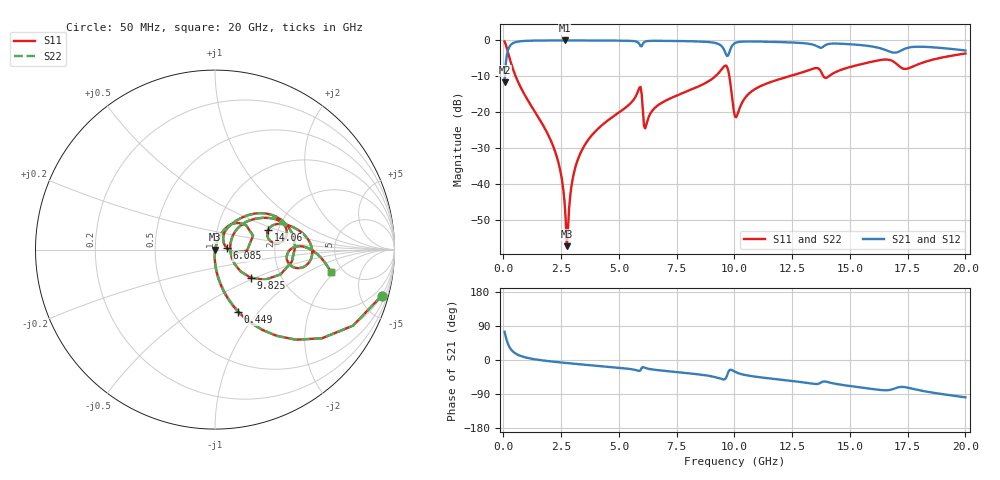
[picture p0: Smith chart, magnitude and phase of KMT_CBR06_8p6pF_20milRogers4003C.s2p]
! Data measured by Modelithics Inc. support@modelithics.com 813-866-6335
! KEMET CBR0603 8.6pF, Pad Width= 0.851mm, Pad Length= 0.64mm, Pad Gap= 0.62mm, 20mil Rogers 4003C substrate Data, January 2022
# hz S ma R 50
! 2 Port Network Data from SP1.SP block
! freq  magS11  angS11  magS21  angS21  magS12  angS12  magS22  angS22
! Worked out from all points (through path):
!   401 points, 50 MHz to 20 GHz, reference 50 ohm
!   highest |S21| = -0.01 dB at 2.643 GHz (marker M1); lowest = -11.6 dB at 50 MHz (marker M2)
!   group delay of S21, straight-line fit = 14.5 ps
!   lowest |S11| = -57.2 dB at 2.743 GHz (marker M3), VSWR 1.00, Z = 50.1 - j0.0686 ohm
!   |S11| at or under -10 dB: 530.9 MHz to 9.169 GHz (8.638 GHz wide, 178 % of centre); 9.781 GHz to 12.35 GHz (2.574 GHz wide, 23.3 % of centre); 13.86 GHz to 14.08 GHz (223.3 MHz wide, 1.6 % of centre)
!   |S22| runs from -57.2 to -0.3 dB; largest |S21 - S12| = 0
!   S11 on the Smith chart (normalised r, x): 50 MHz: 0.98, -7.27; 449 MHz: 0.98, -0.79; 6.085 GHz: 1.14, +0.02; 9.825 GHz: 1.40, -0.47; 14.06 GHz: 1.77, +0.42; 20 GHz: 4.01, -1.79
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5e7  0.9647 -15.4  0.2628 74.6  0.2628 74.6  0.9647 -15.4
2.495e8  0.5893 -54.5  0.8071 35.4  0.8071 35.4  0.5893 -54.5
4.49e8  0.3698 -69.5  0.9282 20.4  0.9282 20.4  0.3698 -69.5
2.194625e9  0.03114 -92.6  0.9983 -4.7  0.9983 -4.7  0.03114 -92.6
2.493875e9  0.01364 -91.4  0.9986 -6.6  0.9986 -6.6  0.01364 -91.4
2.6435e9  0.005742 -84.8  0.9986 -7.5  0.9986 -7.5  0.005742 -84.8
2.74325e9  0.001379 -29.8  0.9986 -8.1  0.9986 -8.1  0.001379 -29.8
3.0425e9  0.01397 74.7  0.9984 -9.8  0.9984 -9.8  0.01397 74.7
3.391625e9  0.02958 75.5  0.998 -11.7  0.998 -11.7  0.02958 75.5
5.8355e9  0.1999 48.0  0.9335 -28.4  0.9335 -28.4  0.1999 48.0
6.084875e9  0.06523 6.7  0.9409 -19.5  0.9409 -19.5  0.06523 6.7
6.73325e9  0.1282 60.7  0.9867 -27.1  0.9867 -27.1  0.1282 60.7
9.276875e9  0.3412 36.3  0.9004 -46.9  0.9004 -46.9  0.3412 36.3
9.626e9  0.4475 2.0  0.6524 -48.3  0.6524 -48.3  0.4475 2.0
9.8255e9  0.2525 -38.2  0.7517 -25.5  0.7517 -25.5  0.2525 -38.2
1.0025e10  0.08737 -9.3  0.918 -31.1  0.918 -31.1  0.08737 -9.3
1.097262e10  0.218 42.4  0.9643 -44.6  0.9643 -44.6  0.218 42.4
1.336662e10  0.4002 22.4  0.88 -62.3  0.88 -62.3  0.4002 22.4
1.406488e10  0.3136 20.0  0.8898 -58.7  0.8898 -58.7  0.3136 20.0
1.670825e10  0.5361 -6.0  0.7025 -79.2  0.7025 -79.2  0.5361 -6.0
1.74065e10  0.4017 -5.0  0.7711 -71.9  0.7711 -71.9  0.4017 -5.0
2e10  0.6579 -11.1  0.7246 -98.6  0.7246 -98.6  0.6579 -11.1
